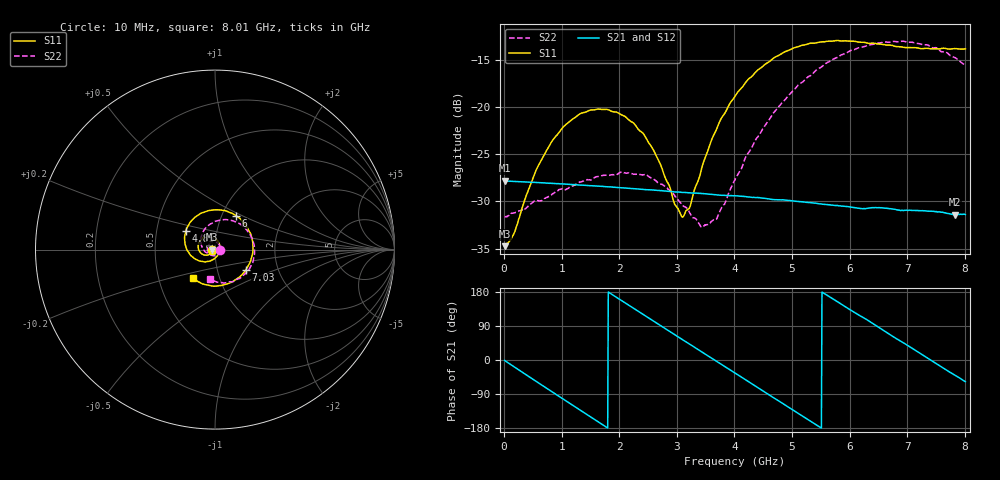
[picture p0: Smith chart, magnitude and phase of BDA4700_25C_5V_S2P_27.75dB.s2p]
!Agilent Technologies,E5071B,MY42404982,A.09.10
!Date: Mon Oct 20 13:40:30 2025
!Data & Calibration Information:
!Freq	S11:SOLT2(ON)	S21:SOLT2(ON)	S12:SOLT2(ON)	S22:SOLT2(ON)
# Hz S RI R 50
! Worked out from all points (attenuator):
!   801 points, 10 MHz to 8.01 GHz, reference 50 ohm
!   highest |S21| = -27.81 dB at 10 MHz (marker M1); lowest = -31.4 dB at 7.83 GHz (marker M2)
!   lowest |S11| = -34.7 dB at 10 MHz (marker M3), VSWR 1.04, Z = 48.2 - j0.0926 ohm
!   |S11| at or under -10 dB: start of sweep to end of sweep
!   |S22| runs from -32.7 to -13.1 dB; largest |S21 - S12| = 0.00035
!   S11 on the Smith chart (normalised r, x): 10 MHz: 0.96, -0.00; 4.85 GHz: 0.71, +0.15; 6 GHz: 1.17, +0.46; 7.03 GHz: 1.37, -0.32; 8.01 GHz: 0.75, -0.25
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1e7  -0.0183 -0.00096  0.0407 -0.000846  0.0406 -0.00091  0.0261 -0.000826
1.6e8  -0.0189 -0.00907  0.0387 -0.0114  0.0387 -0.0115  0.0264 -0.00751
5.4e8  -0.0351 -0.0282  0.0231 -0.0324  0.023 -0.0325  0.0157 -0.0278
7.8e8  -0.0533 -0.031  0.00786 -0.0387  0.00784 -0.0386  0.000371 -0.0335
1.35e9  -0.0927 0.00325  -0.0273 -0.0272  -0.0274 -0.0272  -0.036 -0.0179
2.09e9  -0.0535 0.0715  -0.0329 0.0175  -0.0328 0.0176  -0.0293 0.0339
2.42e9  -0.0126 0.0709  -0.0181 0.0318  -0.018 0.0318  -0.00512 0.0433
2.68e9  0.0142 0.0503  -0.0027 0.036  -0.00275 0.036  0.0127 0.0374
2.97e9  0.0273 0.013  0.0143 0.0324  0.0143 0.0324  0.0256 0.0217
3.12e9  0.0252 -0.00826  0.0219 0.0276  0.0219 0.0277  0.0282 0.0098
3.23e9  0.0195 -0.0224  0.0264 0.0231  0.0265 0.023  0.0273 0.00204
3.54e9  -0.014 -0.0569  0.034 0.00659  0.0339 0.00651  0.0129 -0.02
3.7e9  -0.0405 -0.066  0.0341 -0.00265  0.0342 -0.00273  -0.000515 -0.0259
4.01e9  -0.097 -0.059  0.028 -0.0191  0.0279 -0.0191  -0.0321 -0.0256
4.85e9  -0.1624 0.1053  -0.014 -0.0289  -0.0139 -0.0291  -0.0756 0.0751
5.35e9  -0.0733 0.2042  -0.0299 -0.00844  -0.0299 -0.00848  -0.0153 0.1478
6e9  0.1171 0.1889  -0.0203 0.0215  -0.0205 0.0214  0.131 0.1471
6.68e9  0.2119 -0.00199  0.0103 0.027  0.0104 0.0271  0.2197 0.00101
7.03e9  0.1725 -0.112  0.0229 0.0168  0.0229 0.0167  0.1989 -0.0934
7.45e9  0.0581 -0.1943  0.0279 -0.0021  0.0279 -0.00216  0.1133 -0.1707
7.83e9  -0.0699 -0.1908  0.0206 -0.0173  0.0206 -0.0174  0.0134 -0.1814
8.01e9  -0.1228 -0.1609  0.0145 -0.0227  0.0146 -0.0228  -0.0302 -0.1619
